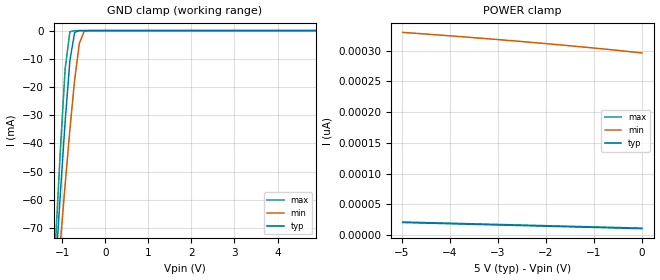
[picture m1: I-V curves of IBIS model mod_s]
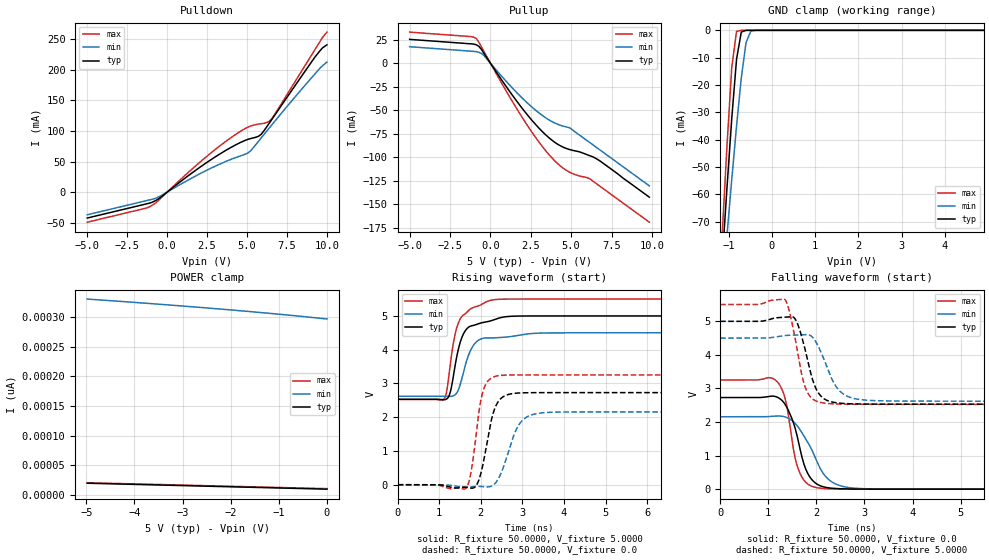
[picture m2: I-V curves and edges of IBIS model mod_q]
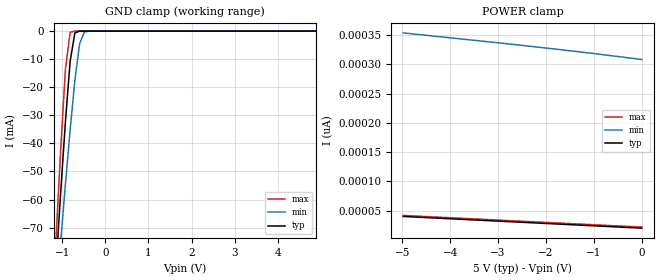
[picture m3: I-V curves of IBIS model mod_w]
| IBIS (I/O, Buffer, Information, Specification) Model, officially
| electronic behavioral standard for Buffer structures of digital pins.
[IBIS ver]  4.0
[File name] m95m02e-a125_5v0_tssop08.ibs
[File Rev]  1.0
[Date]   12 March 2025
[Source]   CAD & Design Services (Catania) - STMicroelectronics
[Notes]
   (Note1)  This IBIS model includes TSSOP8 Package parasitic data
   (Note2)  This IBIS model considers: VCC=5.00(TYP), 4.50(MIN), 5.50(MAX)
   (Note3)  This IBIS model has some Notes about the non-monotonicity
   of the I-V curves, but they are not indicative of problems
   inside the model;
[Disclaimer]
   Customers are solely responsible for all aspects of their
   own product designs or applications using this IBIS Model.
   STMicroelectronics assumes no liability for Custmer Designs
   and applications associated to this IBIS Model.
   In the use of this IBIS Model Customer shall not modify,
   disassemble, alter this Model in whole or in part.
   If Customers do not accept these terms, the IBIS Model
   may not be used. For any problems or modifications please
   contact STMicroelectronics (www.st.com).
[Copyright] (c) 2025 STMicroelectronics
|   Component M95M02E
[Component] M95M02E
[Manufacturer] STMicroelectronics
[Package]
| variable  typ   min   max
R_pkg   0.0   0.0   0.0
L_pkg   0.0H   0.0H   0.0H
C_pkg   0.0F   0.0F   0.0F
[Pin]  signal_name   model_name   R_pin   L_pin   C_pin
1   SN   mod_s   0.0   0.0   0.0
2   Q   mod_q   0.0   0.0   0.0
3   WN   mod_w   0.0   0.0   0.0
4   GND   GND   0.0   0.0   0.0
5   D   mod_d   0.0   0.0   0.0
6   C   mod_c   0.0   0.0   0.0
7   H   mod_h   0.0   0.0   0.0
8   VCC   POWER   0.0   0.0   0.0
[Package Model]  182696_TSSOP8
[Define Package Model]  182696_TSSOP8
[Manufacturer]  STMicroelectronics
[OEM]  STMicroelectronics
[Description]  8 pin TSSOP package
[Number Of Pins]  8
[Pin Numbers]
|Pin Num   Terminal Name
1   | net1
2   | net2
3   | net3
4   | net4_GND
5   | net5
6   | net6
7   | net7
8   | net8_VDD
[Model Data]
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[End Model Data]
[End Package Model]
| Models and submodels in the file (6): mod_s (Input), mod_q (I/O), mod_w (Input), mod_d (Input), mod_c (Input), mod_h (Input)
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|   Model mod_s
[Model]   mod_s
Model_type Input
Vinl   =   1.500V
Vinh   =   3.500V
C_comp   3.207pF   3.063pF   3.358pF
[Temperature Range]  25.0000   0.1250k   -40.0000
[Voltage Range]   5.0000V   4.5000V   5.5000V
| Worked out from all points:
|   GND clamp passes 1 mA (typ) near -0.71 V on its own axis
[GND_clamp]
|Voltage   I(typ)   I(min)   I(max)
-5V       -1.086A    -869.4mA   -1.312A
-1.15V    -83.9mA    -95.64mA   -74.15mA
-1.04V    -57.37mA   -74.82mA   -41.97mA
-930mV    -32.19mA   -54.5mA    -13.5mA
-820mV    -10.62mA   -35.05mA   -415.4uA
-710mV    -636.4uA   -17.42mA   -1.855uA
-600mV    -9.649uA   -4.458mA   -7.81nA
-490mV    -133.7nA   -325.1uA   -35.54pA
-270mV    -27.92pA   -559nA     -546.7fA
4.9V      9.933pA    299.9pA    9.8pA
[POWER_clamp]
|Voltage   I(typ)   I(min)   I(max)
-4.98V    20.14pA    330pA      20.96pA
-4.2V     18.57pA    325.6pA    19.4pA
-3.3V     16.76pA    320.2pA    17.6pA
-2.7V     15.56pA    316.4pA    16.4pA
-1.92V    13.99pA    311.2pA    14.84pA
-900mV    11.94pA    303.8pA    12.8pA
-540mV    11.22pA    301pA      12.08pA
0V        10.13pA    296.5pA    11pA
|   Model mod_q
[Model]   mod_q
Model_type I/O
Polarity   Non-Inverting
Enable   Active-Low
Vinl   =   1.500V
Vinh   =   3.500V
Vmeas  =   2.500V
Cref   =   30pF
C_comp   3.857pF   3.687pF   4.036pF
[Temperature Range]  25.0000   0.1250k   -40.0000
[Voltage Range]   5.0000V   4.5000V   5.5000V
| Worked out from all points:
|   slope of the pulldown table from 0 to 0.75 V, typ, clamps not added: 48.6 ohm
|   slope of the pullup table from 0 to 0.75 V, typ, clamps not added: 39.1 ohm
|   GND clamp passes 1 mA (typ) near -0.71 V on its own axis
|   rising waveform, R_fixture 50.0000, V_fixture 5.0000: 20-80 % time 285ps typ, 309ps min, 281ps max; typ from 2.53 V to 5 V
|   rising waveform, R_fixture 50.0000, V_fixture 0.0: 20-80 % time 272ps typ, 376ps min, 217ps max; typ from 0 V to 2.73 V
|   falling waveform, R_fixture 50.0000, V_fixture 0.0: 20-80 % time 327ps typ, 481ps min, 245ps max; typ from 2.73 V to 0 V
|   falling waveform, R_fixture 50.0000, V_fixture 5.0000: 20-80 % time 280ps typ, 359ps min, 249ps max; typ from 5 V to 2.53 V
[Pulldown]
|Voltage   I(typ)   I(min)   I(max)
-5V       -42.43mA   -37.12mA   -49.24mA
-1V       -17.27mA   -12.12mA   -22.55mA
-520mV    -10.83mA   -7.712mA   -12.98mA
2.84V     54.74mA    40.33mA    66.19mA
4.12V     74.9mA     54.84mA    91.39mA
5.08V     86.54mA    64.45mA    106.6mA
5.88V     94.47mA    88.45mA    111.9mA
6.36V     111.6mA    103.9mA    115.4mA
6.84V     129.9mA    119.2mA    131.8mA
9.24V     220.7mA    193.2mA    232.8mA
9.72V     235.9mA    206.7mA    253.1mA
10V       241mA      212.7mA    261.9mA
[Pullup]
|Voltage   I(typ)   I(min)   I(max)
-5V       25.43mA    17.62mA    33.14mA
-1.2V     20.63mA    12.82mA    28.34mA
-880mV    19.62mA    12.32mA    26.43mA
-720mV    18.03mA    11.68mA    22.47mA
-400mV    10.51mA    8.209mA    12.43mA
2V        -48.7mA    -37.55mA   -58.52mA
2.96V     -68.22mA   -52.24mA   -82.78mA
3.92V     -83.33mA   -63.06mA   -102.7mA
4.88V     -91.69mA   -68.54mA   -115.8mA
6V        -97.41mA   -82.48mA   -121.7mA
6.64V     -102.3mA   -90.48mA   -129.1mA
9.84V     -142.5mA   -130.5mA   -169.1mA
[GND_clamp]
|Voltage   I(typ)   I(min)   I(max)
|Voltage   I(typ)   I(min)   I(max)
-5V       -1.086A    -869.4mA   -1.312A
-1.15V    -83.9mA    -95.64mA   -74.15mA
-1.04V    -57.37mA   -74.82mA   -41.97mA
-930mV    -32.19mA   -54.5mA    -13.5mA
-820mV    -10.62mA   -35.05mA   -415.4uA
-710mV    -636.4uA   -17.42mA   -1.855uA
-600mV    -9.649uA   -4.458mA   -7.81nA
-490mV    -133.7nA   -325.1uA   -35.54pA
-270mV    -27.92pA   -559nA     -546.7fA
4.9V      9.933pA    299.9pA    9.8pA
[POWER_clamp]
|Voltage   I(typ)   I(min)   I(max)
-4.98V    20.14pA    330pA      20.96pA
-4.2V     18.57pA    325.6pA    19.4pA
-3.3V     16.76pA    320.2pA    17.6pA
-2.7V     15.56pA    316.4pA    16.4pA
-1.92V    13.99pA    311.2pA    14.84pA
-900mV    11.94pA    303.8pA    12.8pA
-540mV    11.22pA    301pA      12.08pA
0V        10.13pA    296.5pA    11pA
[Ramp]
| variable   typ   min   max
dV/dt_r   1.6370/0.3122n   1.2939/0.4381n   1.9517/0.2611n
dV/dt_f   1.4813/0.3032n   1.1267/0.3970n   1.7843/0.2875n
R_load = 50.0000
[Rising Waveform]
R_fixture= 50.0000
V_fixture= 5.0000
V_fixture_min= 4.5000
V_fixture_max= 5.5000
|time   V(typ)   V(min)   V(max)
0s        2.532V     2.621V     2.526V
1.11ns    2.518V     2.62V      2.533V
1.19ns    2.552V     2.615V     2.854V
1.27ns    2.765V     2.615V     3.623V
1.37ns    3.451V     2.656V     4.4V
1.49ns    4.163V     2.916V     4.88V
1.63ns    4.57V      3.56V      5.07V
1.81ns    4.715V     4.109V     5.247V
2.23ns    4.852V     4.348V     5.462V
10ns      5V         4.5V       5.5V
[Rising Waveform]
R_fixture= 50.0000
V_fixture= 0.0
V_fixture_min= 0.0
V_fixture_max= 0.0
|time   V(typ)   V(min)   V(max)
0s        1.447nV    2.904uV    245.9pV
1.64ns    -75.41mV   -73.16mV   -108.4mV
1.77ns    -101.6mV   -61.77mV   417mV
1.91ns    19.53mV    -50.12mV   1.733V
2.03ns    485.9mV    -54.34mV   2.671V
2.15ns    1.259V     -65.53mV   3.04V
2.35ns    2.307V     47.38mV    3.211V
2.89ns    2.715V     1.724V     3.253V
3.29ns    2.727V     2.093V     3.253V
10ns      2.728V     2.157V     3.253V
[Falling Waveform]
R_fixture= 50.0000
V_fixture= 0.0
V_fixture_min= 0.0
V_fixture_max= 0.0
|time   V(typ)   V(min)   V(max)
0s        2.728V     2.157V     3.253V
1.2ns     2.732V     2.18V      3.18V
1.36ns    2.507V     2.147V     2.654V
1.54ns    1.91V      1.987V     1.066V
1.62ns    1.468V     1.854V     618.5mV
1.78ns    598.4mV    1.495V     204.2mV
1.98ns    184.7mV    933.6mV    53.77mV
2.28ns    34.87mV    259.5mV    10.15mV
2.8ns     3.299mV    28.26mV    742.1uV
10ns      -5.919nV   2.727uV    23.73nV
[Falling Waveform]
R_fixture= 50.0000
V_fixture= 5.0000
V_fixture_min= 4.5000
V_fixture_max= 5.5000
|time   V(typ)   V(min)   V(max)
0s        5V         4.5V       5.5V
1.34ns    5.121V     4.575V     5.655V
1.42ns    5.128V     4.584V     5.405V
1.56ns    5.069V     4.59V      4.493V
1.76ns    4.199V     4.6V       3.078V
1.94ns    3.182V     4.494V     2.669V
2.1ns     2.765V     4.069V     2.58V
2.44ns    2.569V     3V         2.535V
2.9ns     2.537V     2.671V     2.527V
10ns      2.532V     2.621V     2.526V
|   Model mod_w
[Model]   mod_w
Model_type Input
Vinl   =   1.500V
Vinh   =   3.500V
C_comp   3.207pF   3.063pF   3.358pF
[Temperature Range]  25.0000   0.1250k   -40.0000
[Voltage Range]   5.0000V   4.5000V   5.5000V
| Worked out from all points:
|   GND clamp passes 1 mA (typ) near -0.71 V on its own axis
[GND_clamp]
|Voltage   I(typ)   I(min)   I(max)
-5V       -1.086A    -869.4mA   -1.312A
-1.15V    -83.9mA    -95.65mA   -74.15mA
-1.04V    -57.37mA   -74.82mA   -41.97mA
-930mV    -32.19mA   -54.5mA    -13.5mA
-820mV    -10.62mA   -35.06mA   -419.8uA
-710mV    -639.4uA   -17.42mA   -2.115uA
-600mV    -9.894uA   -4.461mA   -9.088nA
-490mV    -137.6nA   -326.2uA   -42.86pA
-270mV    -29.76pA   -562.6nA   -1.626pA
4.9V      19.79pA    312.3pA    19.6pA
[POWER_clamp]
|Voltage   I(typ)   I(min)   I(max)
-4.98V    40.19pA    353.6pA    41.92pA
-3.36V    33.68pA    339.8pA    35.44pA
-1.98V    28.14pA    327.6pA    29.92pA
-1.08V    24.52pA    319.1pA    26.32pA
0V        20.19pA    308.1pA    22pA
